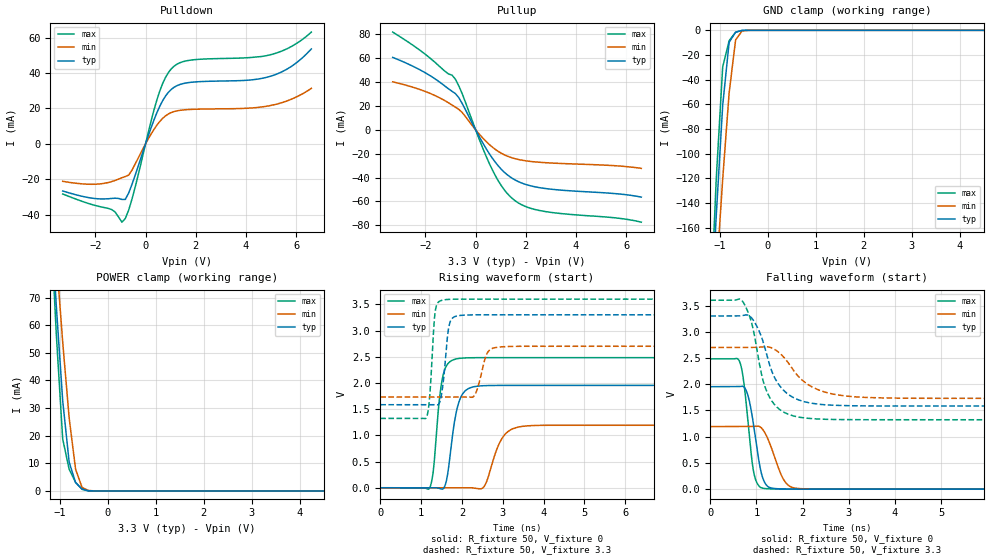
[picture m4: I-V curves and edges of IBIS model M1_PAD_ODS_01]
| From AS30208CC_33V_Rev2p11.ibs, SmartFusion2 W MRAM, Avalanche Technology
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[Model] M1_PAD_ODS_01
Model_type I/O
Enable   Active-High
Vinl  =  0.8
Vinh  =  2.2
Vmeas =  1.65
Cref  =  30e-12
| Capacitance  typ   min   max
C_comp   1.518749e-12   1.424706e-12   1.652746e-12
| Variables   typ   min   max
[GND Clamp Reference]   0   0   0
[POWER Clamp Reference]   3.3   2.7   3.6
[Pulldown Reference]   0   0   0
[Pullup Reference]   3.3   2.7   3.6
[Temperature Range]   25   125   -40
[Voltage Range]   3.3   2.7   3.6
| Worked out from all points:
|   slope of the pulldown table from 0 to 0.495 V, typ, clamps not added: 26.1 ohm
|   slope of the pullup table from 0 to 0.495 V, typ, clamps not added: 27 ohm
|   GND clamp passes 1 mA (typ) near -0.62 V on its own axis
|   POWER clamp passes 1 mA (typ) near -0.56 V on its own axis
|   falling waveform, R_fixture 50, V_fixture 0: 20-80 % time 211ps typ, 305ps min, 176ps max; typ from 1.95 V to 0 V
|   falling waveform, R_fixture 50, V_fixture 3.3: 20-80 % time 457ps typ, 660ps min, 366ps max; typ from 3.3 V to 1.58 V
|   rising waveform, R_fixture 50, V_fixture 0: 20-80 % time 225ps typ, 335ps min, 176ps max; typ from 0 V to 1.95 V
|   rising waveform, R_fixture 50, V_fixture 3.3: 20-80 % time 129ps typ, 193ps min, 104ps max; typ from 1.58 V to 3.3 V
[GND Clamp]
| Voltage   I(typ)   I(min)   I(max)
-3.3V     -1.961A    -1.697A    -2.357A
-1.21V    -250.7mA   -283.7mA   -242.5mA
-1.076V   -150.6mA   -200.1mA   -120.7mA
-941.4mV  -60.83mA   -120.8mA   -29.76mA
-806.9mV  -9.649mA   -50.71mA   -8.442mA
-672.4mV  -1.587mA   -7.866mA   -1.46mA
-537.9mV  -71.93uA   -504.3uA   -18.83uA
-403.4mV  -595.6nA   -18.58uA   -37.45nA
6.6V      0A         0A         0A
[POWER Clamp]
| Voltage   I(typ)   I(min)   I(max)
-3.3V     772.3mA    673.3mA    930.5mA
-1.21V    105.9mA    117.6mA    104.6mA
-1.076V   67.34mA    85.06mA    57.16mA
-941.4mV  32.71mA    53.93mA    18.82mA
-806.9mV  10.48mA    26.53mA    7.848mA
-672.4mV  2.975mA    7.856mA    3.108mA
-537.9mV  710.9uA    1.248mA    573.1uA
-403.4mV  60.69uA    160.8uA    9.187uA
-269mV    142.4nA    6.118uA    23.26nA
6.6V      0A         0A         0A
[Pulldown]
| Voltage   I(typ)   I(min)   I(max)
-3.3V     -26.68mA   -21.22mA   -28.37mA
-1.345V   -30.89mA   -21.35mA   -37.2mA
-941.4mV  -31.46mA   -19.19mA   -44.32mA
-806.9mV  -31.44mA   -18.5mA    -42.21mA
-537.9mV  -22.81mA   -14.83mA   -31.1mA
455.2mV   17.74mA    10.61mA    25.04mA
682.8mV   24.44mA    14.41mA    34.16mA
1.024V    30.75mA    17.67mA    42.38mA
1.821V    34.78mA    19.45mA    47.35mA
4.914V    37.93mA    21.47mA    50.14mA
5.783V    43.54mA    25.06mA    54.82mA
6.6V      53.61mA    31.34mA    63.15mA
[Pullup]
| Voltage   I(typ)   I(min)   I(max)
-3.3V     60.61mA    40.12mA    81.78mA
-1.883V   46.22mA    31.07mA    61.18mA
-806.9mV  30.34mA    18.97mA    42.44mA
-537.9mV  22.21mA    14.55mA    30.44mA
227.6mV   -8.868mA   -5.574mA   -12.38mA
682.8mV   -24.26mA   -14.79mA   -34.2mA
1.138V    -35.44mA   -20.91mA   -50.18mA
1.593V    -42.28mA   -24.34mA   -59.75mA
2.048V    -46.13mA   -26.16mA   -64.77mA
2.731V    -49.08mA   -27.51mA   -68.35mA
5.659V    -53.66mA   -30.27mA   -74.01mA
6.6V      -56.41mA   -32.34mA   -77.42mA
[Ramp]
dV/dt_r   1.17185/0.224543n  0.715782/0.335331n  1.48949/0.176355n
dV/dt_f   1.02933/0.457397n  0.581576/0.659988n  1.3662/0.365774n
R_load = 50
[Falling Waveform]
R_fixture = 50
V_fixture = 0
V_fixture_min = 0
V_fixture_max = 0
| Time   V(typ)   V(min)   V(max)
0s        1.953V     1.193V     2.482V
635.9ps   1.956V     1.193V     2.431V
704.7ps   1.96V      1.193V     2.173V
796.3ps   1.84V      1.193V     1.481V
940.8ps   1.211V     1.196V     323.6mV
1.07ns    457mV      1.192V     48.18mV
1.162ns   158.1mV    1.107V     14.87mV
1.596ns   3.876mV    172.7mV    1.351mV
1.955ns   1.021mV    9.401mV    393uV
21.88ns   -91.88nV   -824.1nV   -402.1nV
[Falling Waveform]
R_fixture = 50
V_fixture = 3.3
V_fixture_min = 2.7
V_fixture_max = 3.6
| Time   V(typ)   V(min)   V(max)
0s        3.3V       2.7V       3.6V
680.8ps   3.304V     2.7V       3.601V
875.3ps   3.282V     2.701V     3.232V
992.1ps   3.135V     2.701V     2.762V
1.133ns   2.84V      2.714V     2.105V
1.288ns   2.362V     2.705V     1.747V
1.59ns    1.883V     2.517V     1.468V
2.081ns   1.658V     2.016V     1.353V
3.936ns   1.585V     1.736V     1.323V
21.88ns   1.584V     1.731V     1.323V
[Rising Waveform]
R_fixture = 50
V_fixture = 0
V_fixture_min = 0
V_fixture_max = 0
| Time   V(typ)   V(min)   V(max)
0s        8.206nV    63.6nV     -79.24nV
1.21ns    786.9uV    36.26uV    -2.765mV
1.297ns   843.1uV    38.84uV    308mV
1.529ns   -24.63mV   45.8uV     2.116V
1.633ns   186.3mV    48.92uV    2.341V
1.918ns   1.614V     57.42uV    2.467V
2.501ns   1.946V     -8.282mV   2.482V
3.016ns   1.953V     981.7mV    2.482V
3.576ns   1.953V     1.179V     2.482V
21.88ns   1.953V     1.193V     2.482V
[Rising Waveform]
R_fixture = 50
V_fixture = 3.3
V_fixture_min = 2.7
V_fixture_max = 3.6
| Time   V(typ)   V(min)   V(max)
0s        1.584V     1.731V     1.323V
1.129ns   1.585V     1.731V     1.34V
1.203ns   1.585V     1.731V     1.679V
1.346ns   1.586V     1.731V     3.368V
1.476ns   1.69V      1.731V     3.568V
1.581ns   2.324V     1.732V     3.588V
1.708ns   3.159V     1.732V     3.595V
2.034ns   3.293V     1.732V     3.599V
2.983ns   3.299V     2.689V     3.599V
21.88ns   3.3V       2.7V       3.6V
